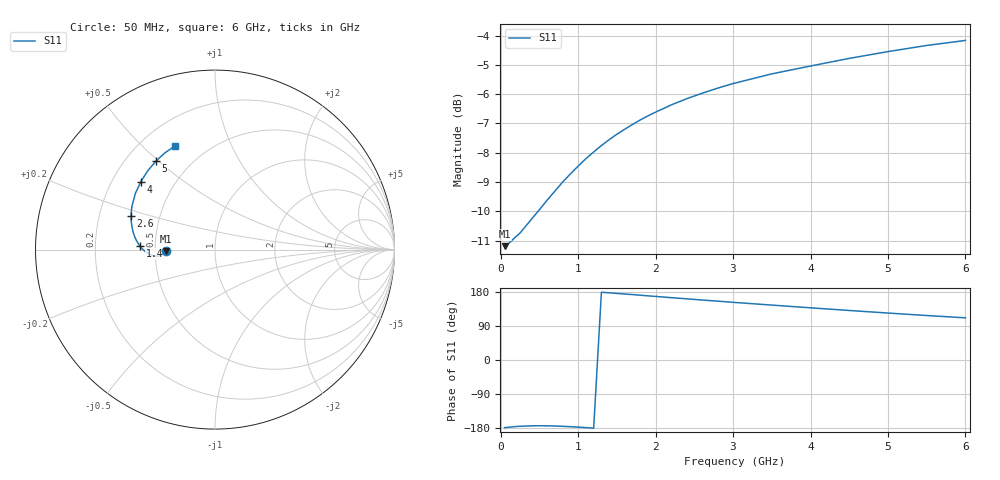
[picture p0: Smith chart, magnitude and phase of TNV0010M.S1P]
! SIEMENS Discrete & RF Semiconductors
! BAS70-07W
! Si Schottky Diode in SOT343
! IF = 10 mA
! S-Parameters:  February  1997
# GHz  S  MA  R  50
!  f  S11
! GHz  MAG  ANG
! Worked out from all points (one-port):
!   34 points, 50 MHz to 6 GHz, reference 50 ohm
!   lowest |S11| = -11.2 dB at 50 MHz (marker M1), VSWR 1.76, Z = 28.4 - j0.444 ohm
!   |S11| at or under -10 dB: start of sweep to 481.6 MHz
!   S11 on the Smith chart (normalised r, x): 50 MHz: 0.57, -0.01; 1.4 GHz: 0.41, +0.02; 2.6 GHz: 0.34, +0.17; 4 GHz: 0.32, +0.35; 5 GHz: 0.32, +0.49; 6 GHz: 0.34, +0.63
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0.05  0.2758 -178.5
0.1  0.2785 -177.4
0.2  0.2866 -175.5
0.25  0.2905 -174.9
0.4  0.307 -173.7
0.5  0.3184 -173.5
0.6  0.3306 -173.7
0.7  0.3425 -174.2
0.8  0.3548 -175.0
1  0.3778 -177.1
1.1  0.389 -178.4
1.3  0.4095 178.8
1.4  0.4191 177.3
1.6  0.4366 174.1
1.8  0.4528 171.0
1.9  0.4601 169.3
2  0.467 167.8
2.2  0.4804 164.5
2.4  0.4923 161.4
2.6  0.503 158.3
2.8  0.5131 155.3
3  0.5225 152.2
3.5  0.5428 144.9
4  0.5598 137.7
4.5  0.5768 130.7
5  0.5925 123.9
5.5  0.6069 117.4
6  0.619 111.3
